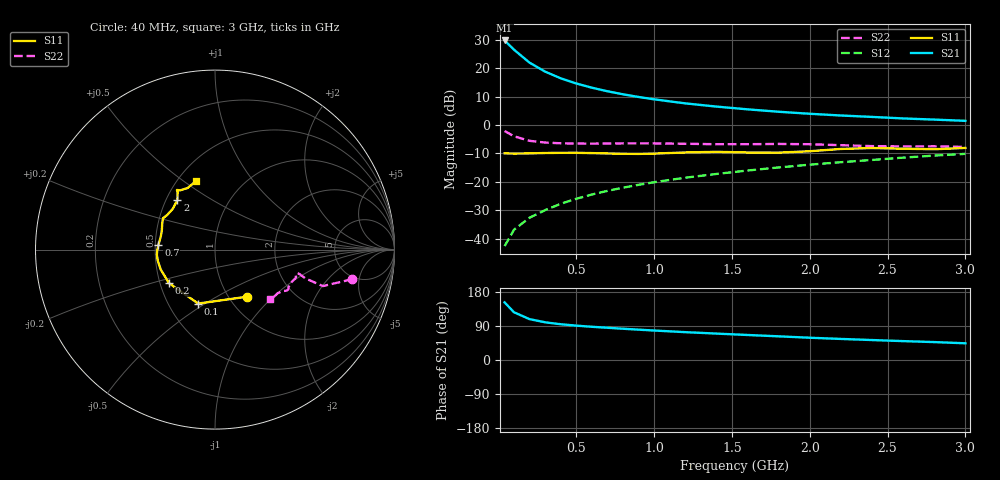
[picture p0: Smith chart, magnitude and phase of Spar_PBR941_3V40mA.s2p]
! Filename:  PBR941I.S2P  Version:  3.0
! NXP part #:  PBR941  Date: July 1998
! Bias condition:  Vce=3V, Ic=40mA
#  MHz  S  MA  R 50
! Freq  S11  S21  S12  S22
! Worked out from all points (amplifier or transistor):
!   21 points, 40 MHz to 3 GHz, reference 50 ohm
!   highest |S21| = 29.7 dB at 40 MHz (marker M1)
!   |S21| within 3 dB of that: start of sweep to 95.6 MHz
!   unconditionally stable (mu >= 1): 151.1 MHz to end of sweep
!   at 300 MHz: K = 1.21, MAG = 21.6 dB, |S12| = -29.9 dB
!   at 1 GHz: K = 1.25, MAG = 11.6 dB, |S12| = -20.1 dB
!   at 3 GHz: K = 1.04, MAG = 4.6 dB, |S12| = -10.1 dB
!   S11 on the Smith chart (normalised r, x): 40 MHz: 1.21, -0.71; 100 MHz: 0.70, -0.47; 200 MHz: 0.56, -0.23; 700 MHz: 0.52, +0.03; 2 GHz: 0.57, +0.36; 3 GHz: 0.62, +0.56
40  0.318 -55.5  30.47 152.0  0.007461 72.3  0.7831 -12.2
100  0.3148 -107.3  20.99 126.0  0.01448 68.9  0.634 -18.7
200  0.3173 -143.8  12.42 107.8  0.02355 71.1  0.5273 -17.6
300  0.3222 -160.0  8.649 99.5  0.03201 74.6  0.4917 -16.2
400  0.3248 -168.8  6.604 94.4  0.0413 76.9  0.4774 -15.9
500  0.3252 -175.2  5.356 90.7  0.05069 79.2  0.4717 -16.2
600  0.3209 -179.9  4.517 87.7  0.06008 79.8  0.4708 -16.8
700  0.3166 175.6  3.915 85.1  0.06973 80.6  0.4725 -17.6
800  0.3123 171.0  3.459 82.5  0.0793 81.1  0.4754 -18.4
900  0.3109 165.4  3.104 80.1  0.08904 81.2  0.4764 -19.1
1000  0.3146 160.5  2.824 77.8  0.09892 81.2  0.4754 -19.8
1200  0.3293 153.2  2.396 73.5  0.1187 80.9  0.468 -21.6
1400  0.3379 148.7  2.105 69.7  0.1381 80.7  0.4599 -24.2
1600  0.329 144.1  1.883 66.0  0.1587 80.2  0.4602 -26.8
1800  0.3271 136.1  1.707 62.5  0.1798 79.6  0.4649 -28.6
2000  0.3461 127.3  1.574 58.8  0.201 78.5  0.4596 -29.9
2200  0.3798 123.2  1.467 55.6  0.2222 77.4  0.4418 -31.6
2400  0.394 122.5  1.386 52.7  0.2433 76.7  0.4256 -34.7
2600  0.3832 120.5  1.303 49.8  0.2674 75.7  0.421 -38.5
2800  0.3755 114.1  1.244 47.3  0.2903 74.3  0.4226 -40.9
3000  0.3954 105.7  1.183 44.1  0.3114 72.8  0.4122 -42.0
